TYPE "ST_AcyclicReadResponse"
VERSION : 0.1


  STRUCT
   byServiceID : BYTE ;	//Sevice ID | Service ID related to the request sent by the client
   dwMessageID : DWORD ;	//Message ID |  Message ID related to the request sent by the client
   dwDataLength : DWORD ;	//Data length | 0x04 (Object index, Sub index, Data type) + data length of the Ob
   byAcknowledge : BYTE ;	//Acknowledge | 0x00 if the access was OK or value unequal 0x00 if not | See ackn
   dwReadType : DWORD ;	//Read type | Read type related to the request sent by the client
   wIndex : WORD ;	//Index | Index of the object to be read
   bySubIndex : BYTE ;	//Sub index | Sub index of the object to be read
   byDataType : BYTE ;	//Data type | Data type of the object to be read
   abyDataByte : ARRAY  [1 .. 76 ] OF //Data bytes | Data bytes of the read value
   BYTE ;
  END_STRUCT ;
END_TYPE

